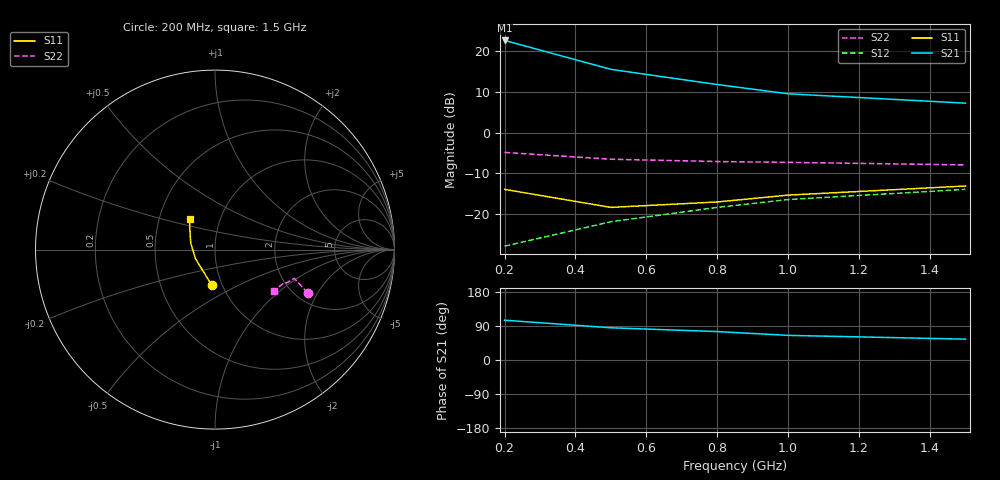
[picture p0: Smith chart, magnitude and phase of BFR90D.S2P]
!  BFR90D.S2P
!  BFR90
!  VCE=5V; IC=20mA
#  GHZ S MA R 50
!  S-PARAMETER DATA
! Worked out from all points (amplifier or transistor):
!   5 points, 200 MHz to 1.5 GHz, reference 50 ohm
!   highest |S21| = 22.7 dB at 200 MHz (marker M1)
!   |S21| within 3 dB of that: start of sweep to 326.6 MHz
!   unconditionally stable (mu >= 1): 614.3 MHz to end of sweep
!   at 200 MHz: K = 0.81, MSG = 25.3 dB, |S12| = -28.0 dB
!   at 800 MHz: K = 1.02, MAG = 14.3 dB, |S12| = -18.4 dB
!   at 1.5 GHz: K = 1.02, MAG = 9.7 dB, |S12| = -14.0 dB
0.2  0.2 -95.0  13.6 105.0  0.04 75.0  0.57 -25.0
0.5  0.12 -155.0  6 85.0  0.08 75.0  0.47 -20.0
0.8  0.14 165.0  3.9 75.0  0.12 75.0  0.44 -25.0
1  0.17 145.0  3 65.0  0.15 70.0  0.43 -25.0
1.5  0.22 130.0  2.3 55.0  0.2 70.0  0.4 -35.0
